(* Logix 5000 AddOnInstructionDefinition export Banner_TL50Pro_PD_v4; software revision 33.00 *)

TYPE Banner_TL50Pro_Adv_PD_Seg_v4 :   // Advanced process data set for a TL50 Pro Segment.
STRUCT
   Segment_Color_1 : SINT;   // 0 = Green, 1 = Red, 2 = Orange, 3 = Amber, 4 = Yellow, 5 = Lime Green, 6 = Spring Green, 7 = Cyan, 8 = Sky Blue, 9 = Blue, 10 = Violet, 11 = Magenta, 12 = Rose, 13 = White, 14 = Custom, 15 = Custom 2
   Segment_Color_1_Intensity : SINT;   // 0 = High, 1 = Low, 2 = Medium, 3 = Off, 4 = Custom
   Segment_Animation_Type : SINT;   // 0 = Off, 1 = Steady, 2 = Flash, 3 = Two Color, 4 = Half/Half, 5 = Half/Half Rotate, 6 = Chase, 7 = Intesnity Sweep
   Segment_Speed : SINT;   // 0 = Medium, 1 = Fast, 2 = Slow, 3 = Custom
   Segment_Pulse_Pattern : SINT;   // 0 = Normal, 1 = Strobe, 2 = Three Pulse, 3 = SOS, 4 = Random
   Segment_Color_2 : SINT;   // 0 = Green, 1 = Red, 2 = Orange, 3 = Amber, 4 = Yellow, 5 = Lime Green, 6 = Spring Green, 7 = Cyan, 8 = Sky Blue, 9 = Blue, 10 = Violet, 11 = Magenta, 12 = Rose, 13 = White, 14 = Custom, 15 = Custom 2
   Segment_Color_2_Instensity : SINT;   // 0 = High, 1 = Low, 2 = Medium, 3 = Off, 4 = Custom
   Segment_Rotational_Direction : SINT;   // 0 = Counter Clockwise, 1 = Clockwise
END_STRUCT
END_TYPE

TYPE Banner_TL50Pro_Adv_PDIO_v4 :   // Advanced process data set for a TL50 Pro IO-Link unit.
STRUCT
   Segment_1 : Banner_TL50Pro_Adv_PD_Seg_v4;   // Advanced process data set for a TL50RGB Segment.
   Segment_2 : Banner_TL50Pro_Adv_PD_Seg_v4;   // Advanced process data set for a TL50RGB Segment.
   Segment_3 : Banner_TL50Pro_Adv_PD_Seg_v4;   // Advanced process data set for a TL50RGB Segment.
   Segment_4 : Banner_TL50Pro_Adv_PD_Seg_v4;   // Advanced process data set for a TL50RGB Segment.
   Segment_5 : Banner_TL50Pro_Adv_PD_Seg_v4;   // Advanced process data set for a TL50RGB Segment.
   Segment_6 : Banner_TL50Pro_Adv_PD_Seg_v4;   // Advanced process data set for a TL50RGB Segment.
   Segment_7 : Banner_TL50Pro_Adv_PD_Seg_v4;   // Advanced process data set for a TL50RGB Segment.
   Segment_8 : Banner_TL50Pro_Adv_PD_Seg_v4;   // Advanced process data set for a TL50RGB Segment.
   Segment_9 : Banner_TL50Pro_Adv_PD_Seg_v4;   // Advanced process data set for a TL50RGB Segment.
   Segment_10 : Banner_TL50Pro_Adv_PD_Seg_v4;   // Advanced process data set for a TL50RGB Segment.
   Audible_State : SINT;   // 0 = Off, 1 = On, 2 = Pulsed, 3 = SOS Pulse
END_STRUCT
END_TYPE

TYPE Banner_TL50Pro_Basic_PD_v4 :   // Basic process data set for a TL50 Pro IO-Link unit.
STRUCT
   Segment_1 : SINT;   // 0 = Off, 1 = On, 2 = Flash, 3 = Animation Type
   Segment_2 : SINT;   // 0 = Off, 1 = On, 2 = Flash, 3 = Animation Type
   Segment_3 : SINT;   // 0 = Off, 1 = On, 2 = Flash, 3 = Animation Type
   Segment_4 : SINT;   // 0 = Off, 1 = On, 2 = Flash, 3 = Animation Type
   Segment_5 : SINT;   // 0 = Off, 1 = On, 2 = Flash, 3 = Animation Type
   Segment_6 : SINT;   // 0 = Off, 1 = On, 2 = Flash, 3 = Animation Type
   Segment_7 : SINT;   // 0 = Off, 1 = On, 2 = Flash, 3 = Animation Type
   Segment_8 : SINT;   // 0 = Off, 1 = On, 2 = Flash, 3 = Animation Type
   Segment_9 : SINT;   // 0 = Off, 1 = On, 2 = Flash, 3 = Animation Type
   Segment_10 : SINT;   // 0 = Off, 1 = On, 2 = Flash, 3 = Animation Type
   Audible_State : SINT;   // 0 = Off, 1 = On, 2 = Pulsed, 3 = SOS Pulse
END_STRUCT
END_TYPE

TYPE Banner_TL50Pro_Level_PD_v4 :   // LeveL process data set for a TL50 Pro IO-Link unit.
STRUCT
   Level_Mode_Value : DINT;   // 0 to 65535. 0 = no lights on while 65535 = all lights on.
   Audible_State : SINT;   // 0 = Off, 1 = On, 2 = Pulsed, 3 = SOS Pulse
END_STRUCT
END_TYPE

TYPE Banner_TL50Pro_PDIO_v4 :   // Process data for a Banner TL50 Pro unit. This includes four process data types.
STRUCT
   Basic_PD : Banner_TL50Pro_Basic_PD_v4;
   Advanced_PD : Banner_TL50Pro_Adv_PDIO_v4;
   Run_PD : Banner_TL50Pro_Run_PD_v4;
   Level_PD : Banner_TL50Pro_Level_PD_v4;
   Transfer_Data : SINT[32];   // Data array to send teh correct state of the process data output to the IO-Link master.
END_STRUCT
END_TYPE

TYPE Banner_TL50Pro_Run_PD_v4 :   // Run mode process data set for a TL50 Pro IO-Link unit.
STRUCT
   Animation : SINT;   // 0 = Off, 1 = Steady, 2 = Flash, 3 = Two Color, 4 = Half/Half, 5 = Half/Half Rotate, 6 = Chase, 7 = Intesnity Sweep, 8 = Scroll, 9 = Bounce, 10 = Demo
   Color_1 : SINT;   // 0 = Green, 1 = Red, 2 = Orange, 3 = Amber, 4 = Yellow, 5 = Lime Green, 6 = Spring Green, 7 = Cyan, 8 = Sky Blue, 9 = Blue, 10 = Violet, 11 = Magenta, 12 = Rose, 13 = White, 14 = Custom, 15 = Custom 2
   Color_1_Intensity : SINT;   // 0 = High, 1 = Low, 2 = Medium, 3 = Off, 4 = Custom
   Speed : SINT;   // 0 = Medium, 1 = Fast, 2 = Slow, 3 = Custom
   Pulse_Pattern : SINT;   // 0 = Normal, 1 = Strobe, 2 = Three Pulse, 3 = SOS, 4 = Random
   Color_2 : SINT;   // 0 = Green, 1 = Red, 2 = Orange, 3 = Amber, 4 = Yellow, 5 = Lime Green, 6 = Spring Green, 7 = Cyan, 8 = Sky Blue, 9 = Blue, 10 = Violet, 11 = Magenta, 12 = Rose, 13 = White, 14 = Custom, 15 = Custom 2
   Color_2_Intensity : SINT;   // 0 = High, 1 = Low, 2 = Medium, 3 = Off, 4 = Custom
   Segement_Shift : SINT;   // 0 = No Shift, 1 = Shift Enabled
   Rotational_Direction : SINT;   // 0 = Counter Clockwise, 1 = Clockwise
   Audible_State : SINT;   // 0 = Off, 1 = On, 2 = Pulsed, 3 = SOS Pulse
END_STRUCT
END_TYPE

ADD_ON_INSTRUCTION Banner_TL50Pro_Adv_PD_v4   (* revision 4.0, vendor Banner Engineering *)
// AOI converts the Advanced process and places it into the correct bytes for transfer to the IO-Link master.
VAR_IN_OUT
   TL50_Pro_Segment : Banner_TL50Pro_Adv_PD_Seg_v4; {required}
   Data_Byte_1 : SINT; {required}
   Data_Byte_2 : SINT; {required}
   Data_Byte_3 : SINT; {required}
END_VAR

ROUTINE Logic   (* ladder *)
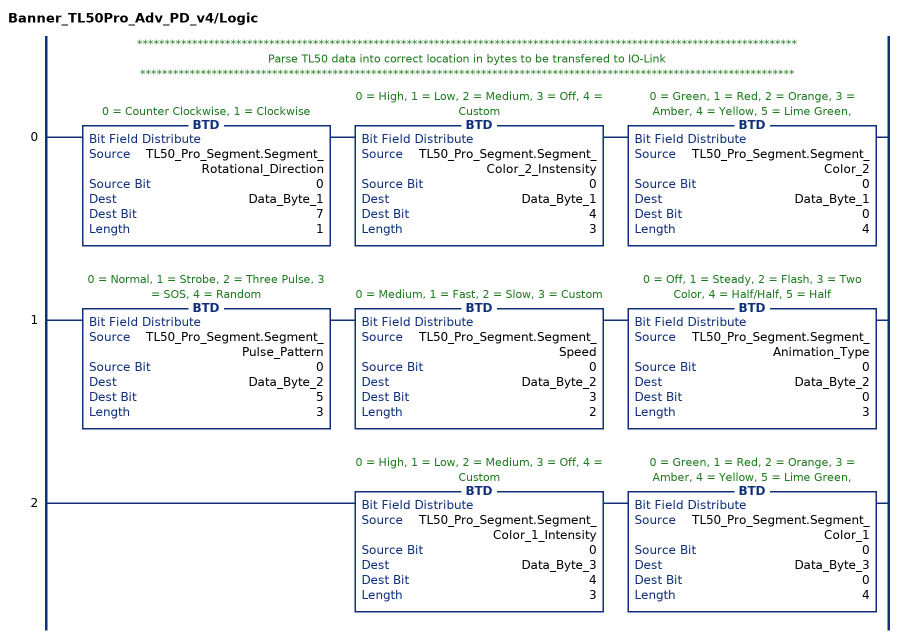
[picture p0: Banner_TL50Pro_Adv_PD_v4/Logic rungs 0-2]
   // ************************************************************************************************************************
   // Parse TL50 data into correct location in bytes to be transfered to IO-Link
   // ***********************************************************************************************************************
   0: BTD(TL50_Pro_Segment.Segment_Rotational_Direction,0,Data_Byte_1,7,1)BTD(TL50_Pro_Segment.Segment_Color_2_Instensity,0,Data_Byte_1,4,3)BTD(TL50_Pro_Segment.Segment_Color_2,0,Data_Byte_1,0,4);
   1: BTD(TL50_Pro_Segment.Segment_Pulse_Pattern,0,Data_Byte_2,5,3)BTD(TL50_Pro_Segment.Segment_Speed,0,Data_Byte_2,3,2)BTD(TL50_Pro_Segment.Segment_Animation_Type,0,Data_Byte_2,0,3);
   2: BTD(TL50_Pro_Segment.Segment_Color_1_Intensity,0,Data_Byte_3,4,3)BTD(TL50_Pro_Segment.Segment_Color_1,0,Data_Byte_3,0,4);
END_ROUTINE
END_ADD_ON_INSTRUCTION

ADD_ON_INSTRUCTION Banner_TL50Pro_PD_v4   (* revision 4.1, vendor Banner Engineering *)
// Takes the raw SINT information and converts that data into actual information.
// Revision note:
// Switched to 32  SINT Array to allow for Byte swap masters.
VAR_IN_OUT
   PROCESS_DATA : Banner_TL50Pro_PDIO_v4; {required}
END_VAR
VAR_INPUT
   Byte_Swap : BOOL; {required}   // Swap the LSB and the MSB with each other.
   Operation_Mode : INT; {required}   // 0 = Basic, 1 = Advanced, 2 = Run, 3 = Level
END_VAR
VAR
   Temp_Measurement : DINT; {access None}
   Data_Byte : SINT[32]; {access None}
   Temp_Data : SINT[32]; {access None}
   AOI_Status : Banner_TL50Pro_Adv_PD_v4[10]; {access None}
END_VAR

ROUTINE Logic   (* ladder *)
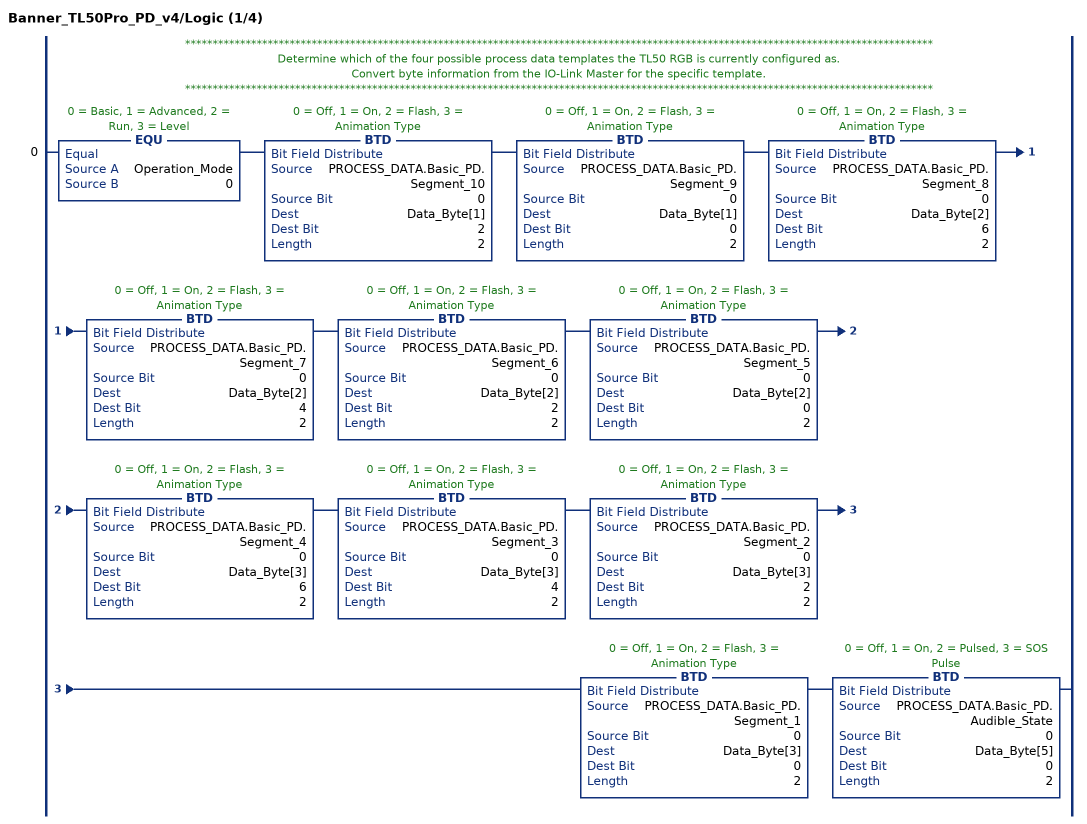
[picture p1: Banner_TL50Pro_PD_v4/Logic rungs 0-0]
   // ****************************************************************************************************************************************
   // Determine which of the four possible process data templates the TL50 RGB is currently configured as.
   // Convert byte information from the IO-Link Master for the specific template.
   // ****************************************************************************************************************************************
   0: EQU(Operation_Mode,0)BTD(PROCESS_DATA.Basic_PD.Segment_10,0,Data_Byte[1],2,2)BTD(PROCESS_DATA.Basic_PD.Segment_9,0,Data_Byte[1],0,2)BTD(PROCESS_DATA.Basic_PD.Segment_8,0,Data_Byte[2],6,2)BTD(PROCESS_DATA.Basic_PD.Segment_7,0,Data_Byte[2],4,2)BTD(PROCESS_DATA.Basic_PD.Segment_6,0,Data_Byte[2],2,2)BTD(PROCESS_DATA.Basic_PD.Segment_5,0,Data_Byte[2],0,2)BTD(PROCESS_DATA.Basic_PD.Segment_4,0,Data_Byte[3],6,2)BTD(PROCESS_DATA.Basic_PD.Segment_3,0,Data_Byte[3],4,2)BTD(PROCESS_DATA.Basic_PD.Segment_2,0,Data_Byte[3],2,2)BTD(PROCESS_DATA.Basic_PD.Segment_1,0,Data_Byte[3],0,2)BTD(PROCESS_DATA.Basic_PD.Audible_State,0,Data_Byte[5],0,2);
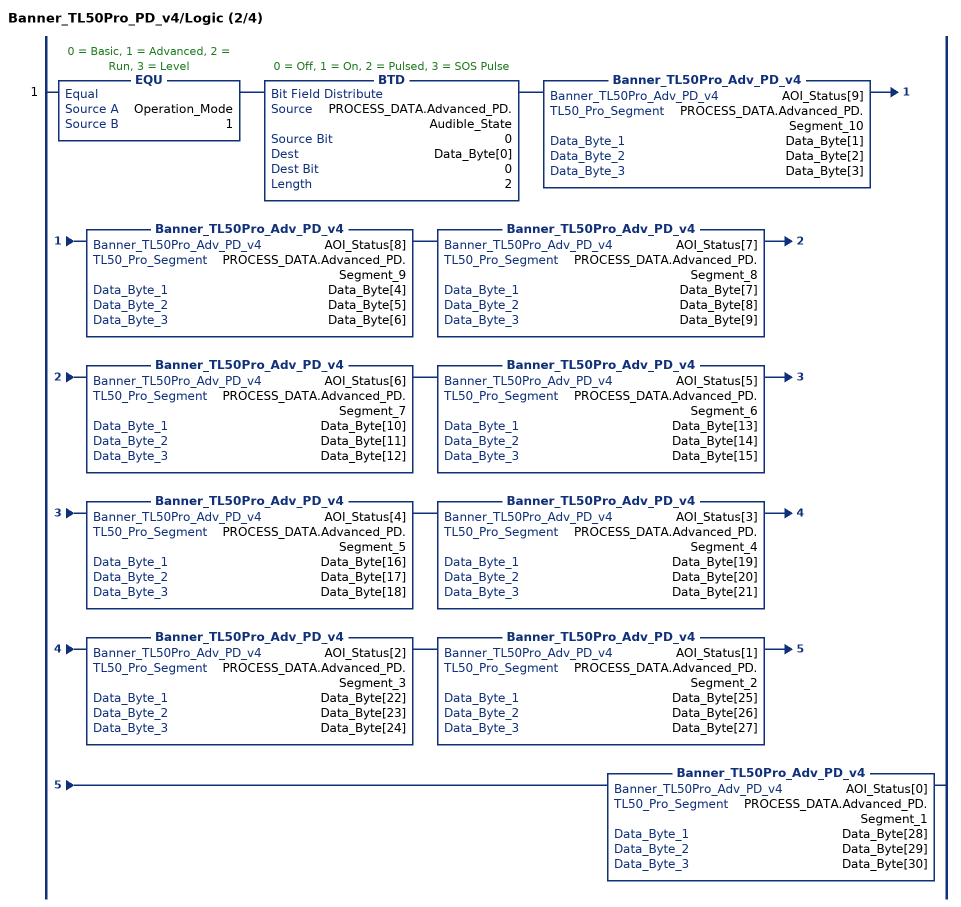
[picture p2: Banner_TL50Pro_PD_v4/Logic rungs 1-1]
   1: EQU(Operation_Mode,1)BTD(PROCESS_DATA.Advanced_PD.Audible_State,0,Data_Byte[0],0,2)Banner_TL50Pro_Adv_PD_v4(AOI_Status[9],PROCESS_DATA.Advanced_PD.Segment_10,Data_Byte[1],Data_Byte[2],Data_Byte[3])Banner_TL50Pro_Adv_PD_v4(AOI_Status[8],PROCESS_DATA.Advanced_PD.Segment_9,Data_Byte[4],Data_Byte[5],Data_Byte[6])Banner_TL50Pro_Adv_PD_v4(AOI_Status[7],PROCESS_DATA.Advanced_PD.Segment_8,Data_Byte[7],Data_Byte[8],Data_Byte[9])Banner_TL50Pro_Adv_PD_v4(AOI_Status[6],PROCESS_DATA.Advanced_PD.Segment_7,Data_Byte[10],Data_Byte[11],Data_Byte[12])Banner_TL50Pro_Adv_PD_v4(AOI_Status[5],PROCESS_DATA.Advanced_PD.Segment_6,Data_Byte[13],Data_Byte[14],Data_Byte[15])Banner_TL50Pro_Adv_PD_v4(AOI_Status[4],PROCESS_DATA.Advanced_PD.Segment_5,Data_Byte[16],Data_Byte[17],Data_Byte[18])Banner_TL50Pro_Adv_PD_v4(AOI_Status[3],PROCESS_DATA.Advanced_PD.Segment_4,Data_Byte[19],Data_Byte[20],Data_Byte[21])Banner_TL50Pro_Adv_PD_v4(AOI_Status[2],PROCESS_DATA.Advanced_PD.Segment_3,Data_Byte[22],Data_Byte[23],Data_Byte[24])Banner_TL50Pro_Adv_PD_v4(AOI_Status[1],PROCESS_DATA.Advanced_PD.Segment_2,Data_Byte[25],Data_Byte[26],Data_Byte[27])Banner_TL50Pro_Adv_PD_v4(AOI_Status[0],PROCESS_DATA.Advanced_PD.Segment_1,Data_Byte[28],Data_Byte[29],Data_Byte[30]);
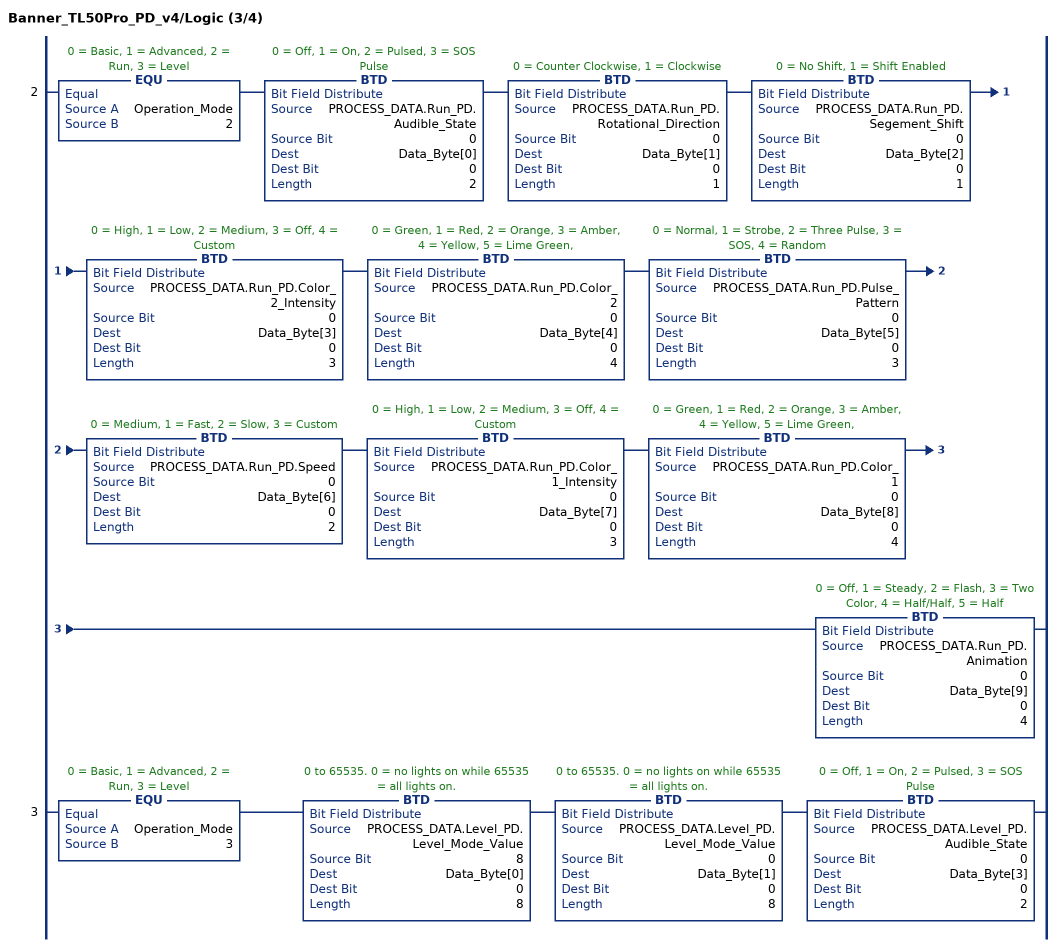
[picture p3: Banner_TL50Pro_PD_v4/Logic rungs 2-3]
   2: EQU(Operation_Mode,2)BTD(PROCESS_DATA.Run_PD.Audible_State,0,Data_Byte[0],0,2)BTD(PROCESS_DATA.Run_PD.Rotational_Direction,0,Data_Byte[1],0,1)BTD(PROCESS_DATA.Run_PD.Segement_Shift,0,Data_Byte[2],0,1)BTD(PROCESS_DATA.Run_PD.Color_2_Intensity,0,Data_Byte[3],0,3)BTD(PROCESS_DATA.Run_PD.Color_2,0,Data_Byte[4],0,4)BTD(PROCESS_DATA.Run_PD.Pulse_Pattern,0,Data_Byte[5],0,3)BTD(PROCESS_DATA.Run_PD.Speed,0,Data_Byte[6],0,2)BTD(PROCESS_DATA.Run_PD.Color_1_Intensity,0,Data_Byte[7],0,3)BTD(PROCESS_DATA.Run_PD.Color_1,0,Data_Byte[8],0,4)BTD(PROCESS_DATA.Run_PD.Animation,0,Data_Byte[9],0,4);
   3: EQU(Operation_Mode,3)BTD(PROCESS_DATA.Level_PD.Level_Mode_Value,8,Data_Byte[0],0,8)BTD(PROCESS_DATA.Level_PD.Level_Mode_Value,0,Data_Byte[1],0,8)BTD(PROCESS_DATA.Level_PD.Audible_State,0,Data_Byte[3],0,2);
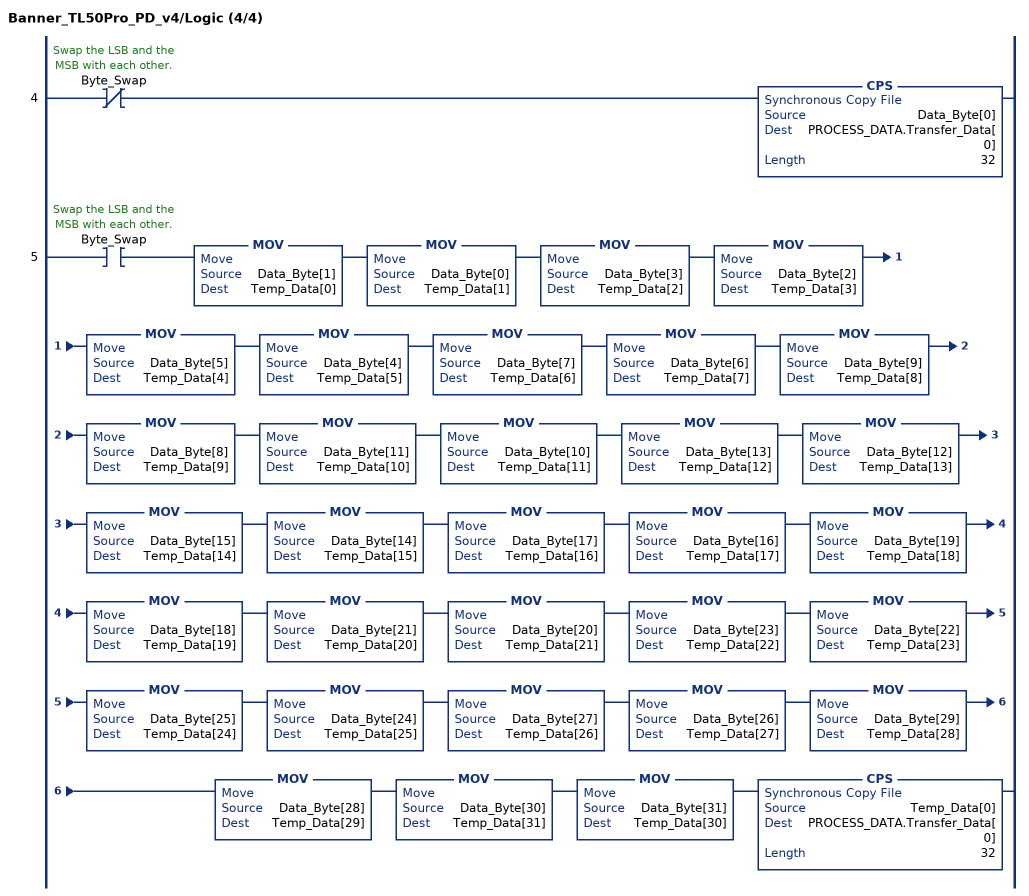
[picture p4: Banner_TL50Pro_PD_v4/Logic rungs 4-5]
   4: XIO(Byte_Swap)CPS(Data_Byte[0],PROCESS_DATA.Transfer_Data[0],32);
   5: XIC(Byte_Swap)MOV(Data_Byte[1],Temp_Data[0])MOV(Data_Byte[0],Temp_Data[1])MOV(Data_Byte[3],Temp_Data[2])MOV(Data_Byte[2],Temp_Data[3])MOV(Data_Byte[5],Temp_Data[4])MOV(Data_Byte[4],Temp_Data[5])MOV(Data_Byte[7],Temp_Data[6])MOV(Data_Byte[6],Temp_Data[7])MOV(Data_Byte[9],Temp_Data[8])MOV(Data_Byte[8],Temp_Data[9])MOV(Data_Byte[11],Temp_Data[10])MOV(Data_Byte[10],Temp_Data[11])MOV(Data_Byte[13],Temp_Data[12])MOV(Data_Byte[12],Temp_Data[13])MOV(Data_Byte[15],Temp_Data[14])MOV(Data_Byte[14],Temp_Data[15])MOV(Data_Byte[17],Temp_Data[16])MOV(Data_Byte[16],Temp_Data[17])MOV(Data_Byte[19],Temp_Data[18])MOV(Data_Byte[18],Temp_Data[19])MOV(Data_Byte[21],Temp_Data[20])MOV(Data_Byte[20],Temp_Data[21])MOV(Data_Byte[23],Temp_Data[22])MOV(Data_Byte[22],Temp_Data[23])MOV(Data_Byte[25],Temp_Data[24])MOV(Data_Byte[24],Temp_Data[25])MOV(Data_Byte[27],Temp_Data[26])MOV(Data_Byte[26],Temp_Data[27])MOV(Data_Byte[29],Temp_Data[28])MOV(Data_Byte[28],Temp_Data[29])MOV(Data_Byte[30],Temp_Data[31])MOV(Data_Byte[31],Temp_Data[30])CPS(Temp_Data[0],PROCESS_DATA.Transfer_Data[0],32);
END_ROUTINE
END_ADD_ON_INSTRUCTION
